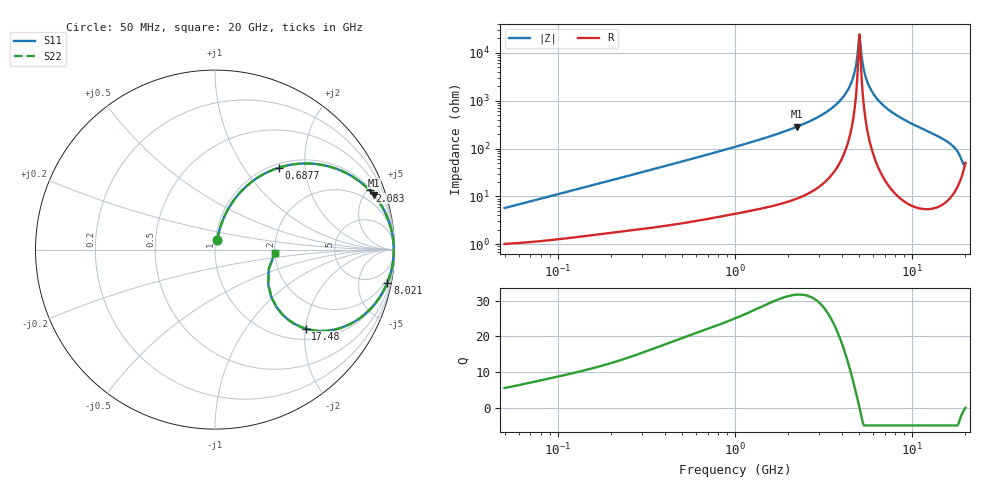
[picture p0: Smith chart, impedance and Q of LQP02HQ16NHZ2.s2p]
!Murata Part Number: LQP02HQ16NHZ2
!These Parameters are Measured in Series Mode Connection
!  o--[Z]--o
!Port1  Port2
!  o-------o
!Freq. Start=50[MHz] Stop=20[GHz], 401[Steps]
# Hz S RI R 50
!Freq.(Hz) S11(Real) S11(Imag) S21(Real) S21(Imag) S12(Real) S12(Imag) S22(Real) S22(Imag)
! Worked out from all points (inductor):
!   401 points, 50 MHz to 20 GHz, reference 50 ohm
!   read as one part in series: L = 17.8 nH near 51.52 MHz
!   highest Q = 31.7 at 2.245 GHz (marker M1), where L = 20.3 nH
!   self-resonance near 5.041 GHz
!   S11 on the Smith chart (normalised r, x): 50 MHz: 1.02, +0.11; 687.7 MHz: 1.07, +1.47; 2.083 GHz: 1.16, +5.15; 8.021 GHz: 1, -10; 17.48 GHz: 1.25, -2.01; 20 GHz: 2.00, -0.08
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5e7  0.0131 0.0549  0.9869 -0.0549  0.9869 -0.0549  0.0131 0.0549
1.364002e8  0.0353 0.1422  0.9647 -0.1422  0.9647 -0.1422  0.0353 0.1422
3.721004e8  0.1511 0.3302  0.8489 -0.3302  0.8489 -0.3302  0.1511 0.3302
6.87656e8  0.3575 0.4571  0.6425 -0.4571  0.6425 -0.4571  0.3575 0.4571
1e9  0.5387 0.4789  0.4613 -0.4789  0.4613 -0.4789  0.5387 0.4789
2.083303e9  0.8615 0.3299  0.1385 -0.3299  0.1385 -0.3299  0.8615 0.3299
2.245319e9  0.8843 0.3045  0.1157 -0.3045  0.1157 -0.3045  0.8843 0.3045
2.728004e9  0.9328 0.2346  0.0672 -0.2346  0.0672 -0.2346  0.9328 0.2346
3.519108e9  0.9745 0.1388  0.0255 -0.1388  0.0255 -0.1388  0.9745 0.1388
4.212059e9  0.9903 0.0699  0.00967 -0.0699  0.00967 -0.0699  0.9903 0.0699
4.608136e9  0.9944 0.0352  0.00561 -0.0352  0.00561 -0.0352  0.9944 0.0352
4.966507e9  0.9958 0.0062  0.00417 -0.0062  0.00417 -0.0062  0.9958 0.0062
5.041459e9  0.9959 0.00038  0.00409 -0.00038  0.00409 -0.00038  0.9959 0.00038
5.194772e9  0.9959 -0.0113  0.00415 0.0113  0.00415 0.0113  0.9959 -0.0113
5.433528e9  0.9952 -0.0288  0.00477 0.0288  0.00477 0.0288  0.9952 -0.0288
5.769027e9  0.9934 -0.0523  0.00661 0.0523  0.00661 0.0523  0.9934 -0.0523
7.442007e9  0.9716 -0.1539  0.0284 0.1539  0.0284 0.1539  0.9716 -0.1539
8.020766e9  0.9604 -0.1844  0.0396 0.1844  0.0396 0.1844  0.9604 -0.1844
1.314879e10  0.7981 -0.3879  0.2019 0.3879  0.2019 0.3879  0.7981 -0.3879
1.747767e10  0.5057 -0.4406  0.4943 0.4406  0.4943 0.4406  0.5057 -0.4406
1.855685e10  0.376 -0.3621  0.624 0.3621  0.624 0.3621  0.376 -0.3621
2e10  0.3336 -0.0169  0.6664 0.0169  0.6664 0.0169  0.3336 -0.0169
